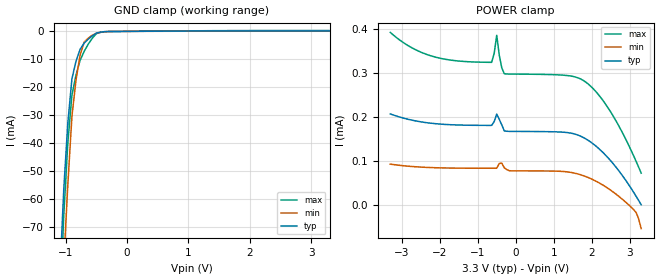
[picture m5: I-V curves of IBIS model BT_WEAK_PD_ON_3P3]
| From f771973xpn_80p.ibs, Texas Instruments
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|   Model Cell BT_WEAK_PD_ON_3P3
|BT_WEAK_PD_ON_3P3
[Model]   BT_WEAK_PD_ON_3P3
Model_type   Input
Polarity   Non-Inverting
Vinl =  0.8
Vinh =  2
C_comp   3.98845p   2.03906p   4.55356p
[Model Spec]
Vinl   0.8   0.8   0.8
Vinh   2   2   2
[Temperature Range]   25   155   -40
[Voltage Range]   3.3   2.97   3.63
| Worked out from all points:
|   GND clamp passes 1 mA (typ) near -0.53 V on its own axis
| Nom Voltages:
|   BIASFET=3.3, VDD=1.2, VDDS=3.3, VSS=0
| Min Voltages:
|   BIASFET=2.97, VDD=1.08, VDDS=2.97, VSS=0
| Max Voltages:
|   BIASFET=3.63, VDD=1.32, VDDS=3.63, VSS=0
[POWER_clamp]
|   voltage   I(typ)   I(min)   I(max)
-3.3V     206.9uA    92.6uA     392.4uA
-2.3V     186.4uA    84.98uA    341uA
-966.7mV  180.9uA    83.25uA    324.7uA
-633.3mV  180.7uA    83.22uA    324.3uA
-566.7mV  189.3uA    83.21uA    344.7uA
-500mV    206.5uA    83.21uA    385.8uA
-366.7mV  181.8uA    94.56uA    311.6uA
-300mV    168uA      84.16uA    298.2uA
1.7V      156.5uA    68.59uA    286.8uA
2.5V      100uA      33.08uA    211uA
3.167V    19.29uA    -17.54uA   98.76uA
3.3V      -340.6pA   -54.3uA    72.05uA
[GND_clamp]
|   voltage   I(typ)   I(min)   I(max)
-3.3V     -1.746A    -1.481A    -2.454A
-1.1V     -88.7mA    -114.8mA   -101.4mA
-1.033V   -56.64mA   -82.93mA   -65.98mA
-966.7mV  -32.73mA   -54.79mA   -39.77mA
-900mV    -16.95mA   -30.37mA   -22.79mA
-833.3mV  -10.65mA   -17.31mA   -15.56mA
-766.7mV  -6.393mA   -8.471mA   -10.34mA
-700mV    -4.19mA    -3.843mA   -7.129mA
-566.7mV  -1.57mA    -1.349mA   -2.424mA
-500mV    -606.7uA   -669.1uA   -790.2uA
-366.7mV  -88.51uA   -120.7uA   -116.4uA
3.3V      167uA      90.89uA    297.2uA
